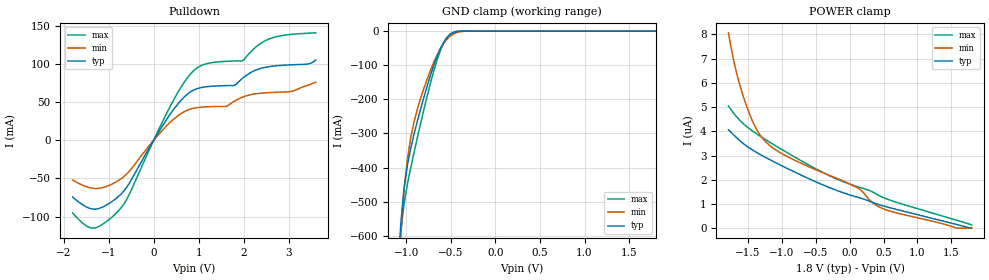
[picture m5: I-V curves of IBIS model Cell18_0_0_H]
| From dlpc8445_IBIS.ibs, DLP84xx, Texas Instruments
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|1I2C ***********************Start I2C 1.8V **********************************
|   Model Cell18_0_0_H
[Model]  Cell18_0_0_H
Model_type I/O_open_drain
Polarity   Non-Inverting
Enable   Active-High
Vinl =  0.540V
Vinh =  1.260V
Vmeas =  0.900V
Cref =  50.000pF
Rref =  1.000M
Vref =  0.0V
C_comp   8.808pF   8.664pF   8.912pF
[Model Spec]
Vinh   1.260V   1.134V   1.386V
Vinl   0.540V   0.486V   0.594V
Vmeas   0.900V   NA   NA
Vref   0.0V   NA   NA
Cref   50.000pF   NA   NA
Rref   1.000M   NA   NA
[Temperature Range]   25.000   0.125k   -40.000
[Voltage Range]   1.800V   1.620V   1.980V
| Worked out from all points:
|   slope of the pulldown table from 0 to 0.27 V, typ, clamps not added: 10.5 ohm
|   GND clamp passes 1 mA (typ) near -0.42 V on its own axis
[Pulldown]
|Voltage   I(typ)   I(min)   I(max)
-1.8V     -74.43mA   -52.12mA   -95.36mA
-1.525V   -86.51mA   -60.23mA   -111.1mA
-1.305V   -90.39mA   -63.27mA   -115.1mA
-755mV    -72.29mA   -51.71mA   -90.8mA
-535mV    -55.85mA   -40.22mA   -70.21mA
400mV     36.93mA    25.37mA    48.14mA
950mV     67.4mA     42.7mA     94.32mA
1.775V    71.64mA    50.63mA    104mA
1.995V    82.32mA    57.1mA     105mA
2.325V    93.33mA    61.41mA    124.9mA
2.655V    97.31mA    62.78mA    134.8mA
3.6V      105.3mA    76.2mA     140.9mA
[GND_clamp]
|Voltage   I(typ)   I(min)   I(max)
-1.8V     -12.3A     -11.29A    -13.31A
-1.097V   -731.7mA   -782.5mA   -731.8mA
-1.06V    -561.7mA   -593mA     -586mA
-1.023V   -458.8mA   -462.4mA   -504.6mA
-986mV    -392.6mA   -374mA     -448.2mA
-912mV    -302.1mA   -266.3mA   -355.6mA
-801mV    -193.6mA   -167.4mA   -229.4mA
-653mV    -73.19mA   -69.93mA   -84.18mA
-579mV    -32.5mA    -36.05mA   -34.84mA
-505mV    -9.454mA   -14.3mA    -8.332mA
-320mV    -34.19uA   -280.6uA   -6.588uA
1.8V      0A         0A         0A
[POWER_clamp]
|Voltage   I(typ)   I(min)   I(max)
-1.789V   4.061uA    8.063uA    5.047uA
-1.678V   3.761uA    6.514uA    4.628uA
-1.604V   3.573uA    5.746uA    4.405uA
-1.493V   3.337uA    4.824uA    4.136uA
-1.345V   3.08uA     3.944uA    3.841uA
-1.16V    2.802uA    3.369uA    3.515uA
-383mV    1.773uA    2.274uA    2.283uA
135mV     1.262uA    1.639uA    1.697uA
320mV     1.081uA    1.1uA      1.523uA
505mV     912.8nA    792nA      1.255uA
1.578V    151.7nA    0A         328nA
1.8V      0A         0A         138.8nA
[Ramp]
| variable   typ   min   max
dV/dt_r   0.891/0.446n   0.740/0.441n   1.022/0.473n
dV/dt_f   0.232/21.132n   91.059m/16.097n   0.455/15.707n
R_load = 50.000
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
